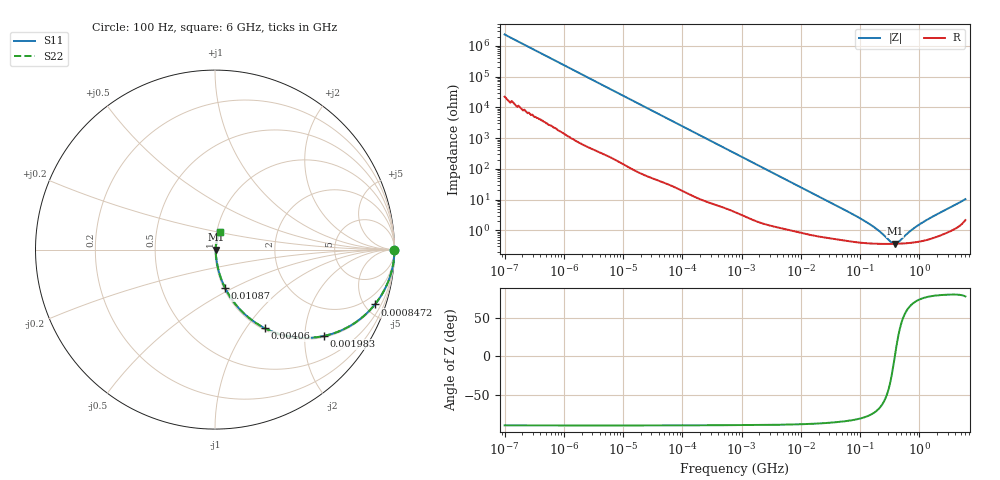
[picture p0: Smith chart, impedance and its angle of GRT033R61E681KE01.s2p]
!Murata Part Number: GRT033R61E681KE01
!These Parameters are Measured in Series Mode Connection
!Data Generated on Jun 19, 2026
!  o--ll--o
!Port1  Port2
!  o------o
!Operation Temp=25[degC], DC Bias Voltage=0[V]
!Freq. Start=100[Hz] Stop=6[GHz] 401[Steps]
# Hz S RI R 50
!Freq.(Hz) S11(Real) S11(Imag) S21(Real) S21(Imag) S12(Real) S12(Imag) S22(Real) S22(Imag)
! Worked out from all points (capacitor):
!   401 points, 100 Hz to 6 GHz, reference 50 ohm
!   read as one part in series: C = 672 pF near 109 Hz
!   lowest |Z| = 364 mohm at 390.8 MHz (marker M1)
!   series resonance near 386.1 MHz, so ESL is about 250 pH
!   S11 on the Smith chart (normalised r, x): 100 Hz: open; 847.2 kHz: 1.07, -5.80; 1.983 MHz: 1.04, -2.49; 4.06 MHz: 1.02, -1.22; 10.87 MHz: 1.02, -0.46; 6 GHz: 1.04, +0.20
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100  1 -4.23e-05  4e-07 4.23e-05  4e-07 4.23e-05  1 -4.23e-05
245  1 -0.000103  7e-07 0.000103  7e-07 0.000103  1 -0.000103
2008  1 -0.00084  5.2e-06 0.00084  5.2e-06 0.00084  1 -0.00084
40335  0.9996 -0.0167  0.000393 0.0167  0.000393 0.0167  0.9996 -0.0167
231233  0.9903 -0.0939  0.00973 0.0939  0.00973 0.0939  0.9903 -0.0939
774597  0.9066 -0.2849  0.0934 0.2849  0.0934 0.2849  0.9066 -0.2849
847162  0.8907 -0.3058  0.1093 0.3058  0.1093 0.3058  0.8907 -0.3058
1267578  0.7877 -0.4024  0.2123 0.4024  0.2123 0.4024  0.7877 -0.4024
1983483  0.6066 -0.4812  0.3934 0.4812  0.3934 0.4812  0.6066 -0.4812
4060267  0.2762 -0.437  0.7238 0.437  0.7238 0.437  0.2762 -0.437
6353432  0.1398 -0.3341  0.8602 0.3341  0.8602 0.3341  0.1398 -0.3341
1.087309e7  0.0573 -0.2157  0.9427 0.2157  0.9427 0.2157  0.0573 -0.2157
1.555665e7  0.0318 -0.1556  0.9682 0.1556  0.9682 0.1556  0.0318 -0.1556
3.64232e7  0.00995 -0.0685  0.99 0.0685  0.99 0.0685  0.00995 -0.0685
1.220122e8  0.00419 -0.0191  0.9958 0.0191  0.9958 0.0191  0.00419 -0.0191
1.996653e8  0.00372 -0.00956  0.9963 0.00956  0.9963 0.00956  0.00372 -0.00956
3.124326e8  0.00361 -0.00288  0.9964 0.00288  0.9964 0.00288  0.00361 -0.00288
3.908258e8  0.00363 0.000167  0.9964 -0.000167  0.9964 -0.000167  0.00363 0.000167
4.470121e8  0.00366 0.00199  0.9963 -0.00199  0.9963 -0.00199  0.00366 0.00199
6.994765e8  0.00395 0.00848  0.996 -0.00848  0.996 -0.00848  0.00395 0.00848
1.094528e9  0.00469 0.0166  0.9953 -0.0166  0.9953 -0.0166  0.00469 0.0166
6e9  0.0306 0.096  0.9694 -0.096  0.9694 -0.096  0.0306 0.096
